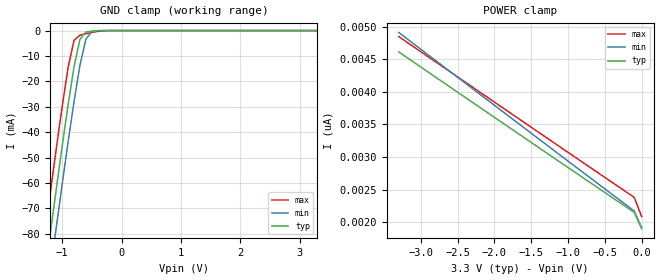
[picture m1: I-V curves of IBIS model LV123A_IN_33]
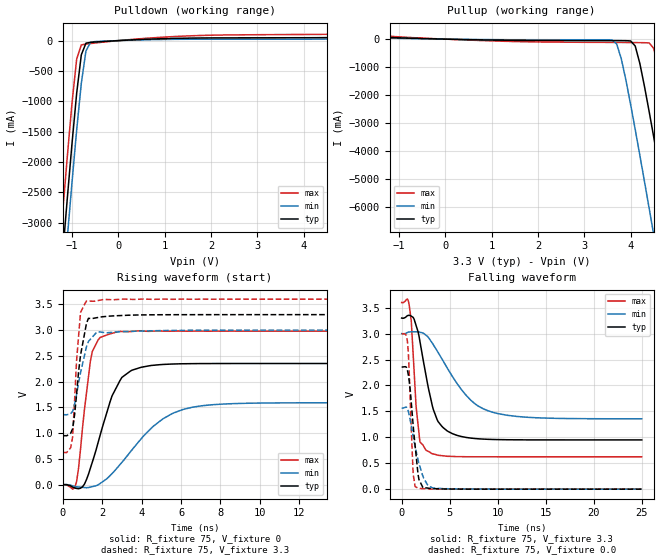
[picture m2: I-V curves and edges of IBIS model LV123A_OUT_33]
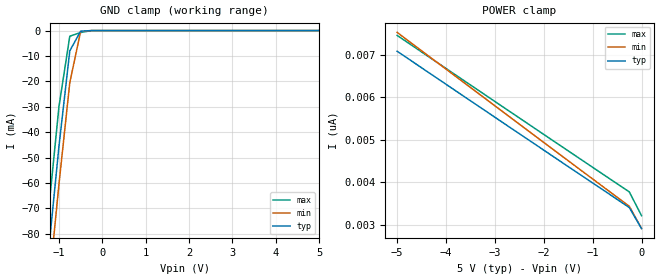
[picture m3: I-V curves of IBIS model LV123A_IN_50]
| TEXAS INSTRUMENTS INCORPORATED
| Standard Linear and Logic Group
| IBIS Model of SN74LV123A
| DUAL RETRIGGERABLE MONOSTABLE MULTIVIBRATORS
| SOIC 16-pin (D), SOP 16-pin (NS), SSOP 16-pin (DB), TSSOP 16-pin (PW)
| and TVSOP 16-pin (DGV) Package
[IBIS Ver]   3.2
[Comment Char]  |_char
[File Name]   lv123a.ibs
[File Rev]   2.0 J_die
[Date]   June 01, 2001
[Source]   Data created from HSPICE simulations at TI-SLL.
[Notes]   The following is an IBIS list for the LV123A.
|   Please contact sllibis@ti.com with questions and
|   comments concerning SLL IBIS models.
[Disclaimer] Property of Texas Instruments Incorporated.  Unauthorized
   reproduction and/or distribution is strictly prohibited.
   This product is protected under copyright law.
   Created 2001, (C) Copyright 2001, Texas Instruments Inc.,
   All Rights Reserved.
   UNLESS THERE IS A SIGNED, WRITTEN AGREEMENT TO THE
   CONTRARY, TEXAS INSTRUMENTS ("TI") IS PROVIDING THE IBIS
   MODELS "AS IS" AND WITHOUT ANY WARRANTY, EXPRESSED OR
   IMPLIED.  TI assumes no liability for:
   1) the accuracy of the IBIS models provided to your
   company;
   2) the proper functioning of these IBIS Models in your
   design or for any resulting applications; or
   3) infringement of patents, copyrights or intellectual
   property rights resulting from your use of these IBIS
   models.
   TI provides IBIS Models as a service to our customers.
   You and your company shall not distribute, sell or give
   these models to anyone else without prior written
   permission from TI.
   TI reserves the right to make changes to our products or
   to discontinue any semiconductor product or service
   without notice, and advises our customers to obtain the
   latest version of relevant information to verify, before
   placing orders, that the information being relied on is
   current.
   Please be aware that your receipt and use of the IBIS
   information provided shall serve as acceptance of these
   terms and conditions.  If you do not accept these terms,
   you should return or destroy the IBIS models and any
   other accompanying information immediately.
|   Component LV123A_D
[Component]   LV123A_D
[Manufacturer]  Texas Instruments, Inc.
[Package]
|   typ   min   max
R_pkg   0.039   0.028   0.049
L_pkg   3.453nH   2.350nH   4.375nH
C_pkg   0.521pF   0.254pF   0.708pF
[Pin]   signal_name   model_name   R_pin   L_pin   C_pin
1   1A_NOT   LV123A_IN   0.042   4.336nH   0.703pF
2   1B   LV123A_IN   0.049   3.778nH   0.634pF
3   1CLR_NOT   LV123A_IN   0.028   3.449nH   0.518pF
4   1Q_NOT   LV123A_OUT   0.029   2.393nH   0.254pF
5   2Q   LV123A_OUT   0.028   2.350nH   0.264pF
6   2Cext   LV123A_IN   0.048   3.312nH   0.483pF
7   2Rext_or_Cext   LV123A_IN   0.043   3.629nH   0.604pF
8   GND   GND   0.044   4.375nH   0.708pF
9   2A_NOT   LV123A_IN   0.042   4.336nH   0.703pF
10   2B   LV123A_IN   0.049   3.778nH   0.634pF
11   2CLR_NOT   LV123A_IN   0.028   3.449nH   0.518pF
12   2Q_NOT   LV123A_OUT   0.029   2.393nH   0.255pF
13   1Q   LV123A_OUT   0.028   2.350nH   0.264pF
14   1Cext   LV123A_IN   0.048   3.312nH   0.483pF
15   1Rext_or_Cext   LV123A_IN   0.043   3.629nH   0.604pF
16   VCC   POWER   0.044   4.375nH   0.708pF
|   Component LV123A_NS
[Component]   LV123A_NS
[Manufacturer]  Texas Instruments, Inc.
[Package]
|   typ   min   max
R_pkg   0.042   0.035   0.049
L_pkg   3.147nH   2.164nH   4.219nH
C_pkg   0.404pF   0.241pF   0.562pF
[Pin]   signal_name   model_name   R_pin   L_pin   C_pin
1   1A_NOT   LV123A_IN   0.049   4.215nH   0.562pF
2   1B   LV123A_IN   0.046   3.675nH   0.480pF
3   1CLR_NOT   LV123A_IN   0.037   2.527nH   0.332pF
4   1Q_NOT   LV123A_OUT   0.035   2.164nH   0.241pF
5   2Q   LV123A_OUT   0.035   2.164nH   0.241pF
6   2Cext   LV123A_IN   0.037   2.527nH   0.332pF
7   2Rext_or_Cext   LV123A_IN   0.046   3.675nH   0.480pF
8   GND   GND   0.049   4.215nH   0.562pF
9   2A_NOT   LV123A_IN   0.049   4.219nH   0.562pF
10   2B   LV123A_IN   0.046   3.679nH   0.480pF
11   2CLR_NOT   LV123A_IN   0.037   2.531nH   0.333pF
12   2Q_NOT   LV123A_OUT   0.035   2.168nH   0.241pF
13   1Q   LV123A_OUT   0.035   2.168nH   0.241pF
14   1Cext   LV123A_IN   0.037   2.531nH   0.333pF
15   1Rext_or_Cext   LV123A_IN   0.046   3.679nH   0.480pF
16   VCC   POWER   0.049   4.219nH   0.562pF
|   Component LV123A_DB
[Component]   LV123A_DB
[Manufacturer]  Texas Instruments, Inc.
[Package]
|   typ   min   max
R_pkg   0.048   0.046   0.050
L_pkg   3.536nH   3.213nH   3.798nH
C_pkg   0.376pF   0.314pF   0.440pF
[Pin]   signal_name   model_name   R_pin   L_pin   C_pin
1   1A_NOT   LV123A_IN   0.048   3.797nH   0.377pF
2   1B   LV123A_IN   0.046   3.723nH   0.440pF
3   1CLR_NOT   LV123A_IN   0.048   3.409nH   0.372pF
4   1Q_NOT   LV123A_OUT   0.049   3.213nH   0.314pF
5   2Q   LV123A_OUT   0.049   3.213nH   0.314pF
6   2Cext   LV123A_IN   0.048   3.409nH   0.372pF
7   2Rext_or_Cext   LV123A_IN   0.046   3.723nH   0.440pF
8   GND   GND   0.048   3.798nH   0.377pF
9   2A_NOT   LV123A_IN   0.048   3.797nH   0.377pF
10   2B   LV123A_IN   0.046   3.725nH   0.440pF
11   2CLR_NOT   LV123A_IN   0.048   3.409nH   0.372pF
12   2Q_NOT   LV123A_OUT   0.049   3.214nH   0.314pF
13   1Q   LV123A_OUT   0.050   3.216nH   0.314pF
14   1Cext   LV123A_IN   0.048   3.409nH   0.372pF
15   1Rext_or_Cext   LV123A_IN   0.047   3.729nH   0.440pF
16   VCC   POWER   0.048   3.797nH   0.377pF
|   Component LV123A_PW
[Component]   LV123A_PW
[Manufacturer]  Texas Instruments, Inc.
[Package]
|   typ   min   max
R_pkg   0.045   0.038   0.051
L_pkg   2.593nH   2.447nH   3.080nH
C_pkg   0.281pF   0.243pF   0.377pF
[Pin]   signal_name   model_name   R_pin   L_pin   C_pin
1   1A_NOT   LV123A_IN   0.040   3.080nH   0.377pF
2   1B   LV123A_IN   0.038   2.458nH   0.281pF
3   1CLR_NOT   LV123A_IN   0.051   2.512nH   0.255pF
4   1Q_NOT   LV123A_OUT   0.051   2.447nH   0.243pF
5   2Q   LV123A_OUT   0.051   2.447nH   0.243pF
6   2Cext   LV123A_IN   0.051   2.512nH   0.255pF
7   2Rext_or_Cext   LV123A_IN   0.038   2.458nH   0.281pF
8   GND   GND   0.040   3.080nH   0.377pF
9   2A_NOT   LV123A_IN   0.039   2.832nH   0.316pF
10   2B   LV123A_IN   0.038   2.460nH   0.279pF
11   2CLR_NOT   LV123A_IN   0.051   2.512nH   0.255pF
12   2Q_NOT   LV123A_OUT   0.051   2.447nH   0.243pF
13   1Q   LV123A_OUT   0.051   2.447nH   0.243pF
14   1Cext   LV123A_IN   0.051   2.512nH   0.255pF
15   1Rext_or_Cext   LV123A_IN   0.038   2.459nH   0.279pF
16   VCC   POWER   0.039   2.832nH   0.316pF
|   Component LV123A_DGV
[Component]   LV123A_DGV
[Manufacturer]  Texas Instruments, Inc.
[Package]
|   typ   min   max
R_pkg   0.039   0.033   0.045
L_pkg   2.543nH   2.320nH   2.938nH
C_pkg   0.386pF   0.334pF   0.449pF
[Pin]   signal_name   model_name   R_pin   L_pin   C_pin
1   1A_NOT   LV123A_IN   0.035   2.907nH   0.417pF
2   1B   LV123A_IN   0.042   2.558nH   0.446pF
3   1CLR_NOT   LV123A_IN   0.038   2.341nH   0.345pF
4   1Q_NOT   LV123A_OUT   0.038   2.320nH   0.334pF
5   2Q   LV123A_OUT   0.039   2.322nH   0.334pF
6   2Cext   LV123A_IN   0.038   2.353nH   0.342pF
7   2Rext_or_Cext   LV123A_IN   0.040   2.536nH   0.441pF
8   GND   GND   0.033   2.897nH   0.418pF
9   2A_NOT   LV123A_IN   0.035   2.927nH   0.419pF
10   2B   LV123A_IN   0.045   2.632nH   0.449pF
11   2CLR_NOT   LV123A_IN   0.039   2.368nH   0.347pF
12   2Q_NOT   LV123A_OUT   0.039   2.330nH   0.335pF
13   1Q   LV123A_OUT   0.039   2.320nH   0.335pF
14   1Cext   LV123A_IN   0.039   2.361nH   0.345pF
15   1Rext_or_Cext   LV123A_IN   0.041   2.573nH   0.446pF
16   VCC   POWER   0.035   2.938nH   0.420pF
[Model Selector]   LV123A_IN
LV123A_IN_33   3.3-V Vcc Input Model
LV123A_IN_50   5.0-V Vcc Input Model
[Model Selector]   LV123A_OUT
LV123A_OUT_33   3.3-V Vcc Output Model
LV123A_OUT_50   5.0-V Vcc Output Model
| Models and submodels in the file (4): LV123A_IN_33 (Input), LV123A_OUT_33 (Output), LV123A_IN_50 (Input), LV123A_OUT_50 (Output)
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|   Model LV123A_IN_33
[Model]   LV123A_IN_33
Model_type  Input
Polarity   Inverting
Vinl = 0.99
Vinh = 2.31
| variable   typ   min   max
C_comp   1.49pf   1.12pf   1.86pf
[Temperature Range]   25   85   -40
[Voltage Range]   3.3   3.0   3.6
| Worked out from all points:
|   GND clamp passes 1 mA (typ) near -0.61 V on its own axis
[GND Clamp]
|   Voltage   I(typ)   I(min)   I(max)
-3.3V     -460.4mA   -474.6mA   -445.4mA
-1.3V     -97.49mA   -112.5mA   -81.51mA
-1.2V     -79.93mA   -94.98mA   -63.94mA
-1.1V     -62.59mA   -77.62mA   -46.67mA
-1V       -45.6mA    -60.54mA   -29.97mA
-900mV    -29.25mA   -43.87mA   -14.58mA
-800mV    -14.28mA   -27.95mA   -3.811mA
-700mV    -3.418mA   -13.61mA   -1.784mA
-600mV    -581.1uA   -3.398mA   -1.247mA
-500mV    -232.6uA   -352.5uA   -758.6uA
-400mV    -58.12uA   -21.94uA   -324.1uA
3.3V      1.902nA    2.343nA    1.692nA
[POWER Clamp]
|   Voltage   I(typ)   I(min)   I(max)
-3.3V     4.612nA    4.91nA     4.847nA
-1.6V     3.301nA    3.451nA    3.534nA
-100mV    2.151nA    2.173nA    2.382nA
0V        1.902nA    1.921nA    2.089nA
|   Model LV123A_OUT_33
[Model]   LV123A_OUT_33
Model_type  Output
Polarity   Non-Inverting
Vmeas = 1.65v
Cref = 15pf
| variable   typ   min   max
C_comp   4.62pf   3.47pf   5.77pf
[Temperature Range]   25   85   -40
[Voltage Range]   3.3   3.0   3.6
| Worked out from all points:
|   slope of the pulldown table from 0 to 0.495 V, typ, clamps not added: 26.1 ohm
|   slope of the pullup table from 0 to 0.495 V, typ, clamps not added: 27.2 ohm
|   rising waveform, R_fixture 75, V_fixture 0: 20-80 % time 1.19ns typ, 2.33ns min, 522ps max; typ from 0 V to 2.35 V
|   falling waveform, R_fixture 75, V_fixture 3.3: 20-80 % time 1.61ns typ, 3.71ns min, 646ps max; typ from 3.3 V to 0.95 V
|   rising waveform, R_fixture 75, V_fixture 3.3: 20-80 % time 440ps typ, 533ps min, 287ps max; typ from 0.95 V to 3.3 V
|   falling waveform, R_fixture 75, V_fixture 0.0: 20-80 % time 697ps typ, 1.13ns min, 376ps max; typ from 2.36 V to 0 V
[Pulldown]
|   Voltage   I(typ)   I(min)   I(max)
-3.3V     -24A       -24.6A     -23.38A
-1.3V     -4.436A    -5.085A    -3.748A
-1.2V     -3.498A    -4.148A    -2.807A
-1.1V     -2.577A    -3.226A    -1.889A
-1V       -1.688A    -2.327A    -1.02A
-900mV    -865.4mA   -1.471A    -303.5mA
-800mV    -234mA     -703.4mA   -70.75mA
-700mV    -41.6mA    -170.5mA   -56.88mA
-600mV    -28.42mA   -27.34mA   -48.15mA
-400mV    -18.31mA   -11.94mA   -30.69mA
1.5V      40.71mA    22.55mA    77.22mA
6.6V      95.54mA    55.18mA    175.9mA
[Pullup]
|   Voltage   I(typ)   I(min)   I(max)
-3.3V     176.8mA    99.77mA    326.3mA
3.6V      -52.86mA   -33.07mA   -117.3mA
3.7V      -53.3mA    -173.1mA   -117.9mA
3.8V      -54.21mA   -704.2mA   -118.5mA
4.1V      -245.8mA   -3.226A    -123mA
4.2V      -869.9mA   -4.148A    -125.5mA
4.4V      -2.579A    -6.032A    -134.7mA
4.5V      -3.499A    -6.986A    -333mA
4.8V      -6.344A    -9.879A    -2.811A
4.9V      -7.308A    -10.85A    -3.751A
5.2V      -10.22A    -13.78A    -6.633A
6.6V      -24A       -27.56A    -20.4A
[Ramp]
| variable   typ   min   max
dV/dt_r  1.4179E+00/1.1422E-09  9.6900E-01/2.3888E-09  1.7956E+00/5.1105E-10
dV/dt_f  1.4424E+00/1.5998E-09  1.0078E+00/3.7515E-09  1.8270E+00/6.1666E-10
R_load = 75
[Rising Waveform]
R_fixture = 75
V_fixture = 0
|   Time   V(typ)   V(min)   V(max)
0s        0V         0V         0V
700ps     -71.18mV   -39.38mV   60.11mV
1.1ns     13.5mV     -53.76mV   1.461V
1.5ns     440.4mV    -36.37mV   2.588V
2.4ns     1.61V      178mV      2.927V
3ns       2.083V     434.7mV    2.973V
3.5ns     2.221V     671.4mV    2.974V
5.1ns     2.334V     1.283V     2.981V
6.6ns     2.349V     1.506V     2.98V
25ns      2.352V     1.591V     2.98V
[Falling Waveform]
R_fixture = 75
V_fixture = 3.3
V_fixture_min = 3.0
V_fixture_max = 3.6
|   Time   V(typ)   V(min)   V(max)
0s        3.3V       3V         3.6V
800ps     3.353V     3.032V     3.53V
1ns       3.336V     3.034V     3.247V
1.5ns     3.159V     3.035V     1.602V
1.9ns     2.853V     3.027V     914.8mV
2.6ns     2.128V     2.959V     742.7mV
3.3ns     1.536V     2.785V     678.5mV
4.3ns     1.19V      2.478V     644mV
9ns       961.4mV    1.512V     624.2mV
25ns      950mV      1.357V     624mV
[Rising Waveform]
R_fixture = 75
V_fixture = 3.3
V_fixture_min = 3.0
V_fixture_max = 3.6
|   Time   V(typ)   V(min)   V(max)
0s        950mV      1.357V     624mV
400ps     997.8mV    1.377V     718.1mV
500ps     1.087V     1.424V     925.5mV
700ps     1.749V     1.752V     2.408V
800ps     2.189V     1.976V     2.875V
900ps     2.512V     2.172V     3.341V
1.2ns     3.127V     2.674V     3.565V
1.3ns     3.228V     2.779V     3.563V
1.8ns     3.246V     2.969V     3.574V
25ns      3.3V       3V         3.6V
[Falling Waveform]
R_fixture = 75
V_fixture = 0.0
|   Time   V(typ)   V(min)   V(max)
0s        2.357V     1.563V     2.996V
600ps     2.296V     1.557V     2.852V
700ps     2.2V       1.499V     2.624V
1.2ns     1.227V     1.012V     290.2mV
1.4ns     842mV      829.3mV    51.37mV
1.8ns     185.8mV    495.6mV    17.84mV
2.3ns     18.42mV    209.2mV    9.892mV
2.8ns     18.08mV    60.21mV    4.533mV
4.2ns     4.139mV    11.36mV    1.475mV
25ns      0V         1.047uV    5.72uV
|   Model LV123A_IN_50
[Model]   LV123A_IN_50
Model_type  Input
Polarity   Inverting
Vinl = 1.5
Vinh = 3.5
| variable   typ   min   max
C_comp   1.49pf   1.12pf   1.86pf
[Temperature Range]   25   85   -40
[Voltage Range]   5.0   4.5   5.5
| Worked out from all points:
|   GND clamp passes 1 mA (typ) near -0.52 V on its own axis
[GND Clamp]
|   Voltage   I(typ)   I(min)   I(max)
-5V       -772.7mA   -786.5mA   -758.1mA
-1.5V     -133mA     -148mA     -117.2mA
-1.25V    -88.68mA   -103.7mA   -72.7mA
-1V       -45.6mA    -60.54mA   -29.97mA
-750mV    -7.993mA   -20.49mA   -2.232mA
-500mV    -232.6uA   -352.5uA   -758.6uA
-250mV    -2.633nA   -182.1nA   -26.9uA
5V        2.904nA    3.644nA    2.541nA
[POWER Clamp]
|   Voltage   I(typ)   I(min)   I(max)
-5V       7.079nA    7.524nA    7.452nA
-2.5V     5.139nA    5.363nA    5.509nA
-250mV    3.401nA    3.43nA     3.769nA
0V        2.904nA    2.91nA     3.209nA
